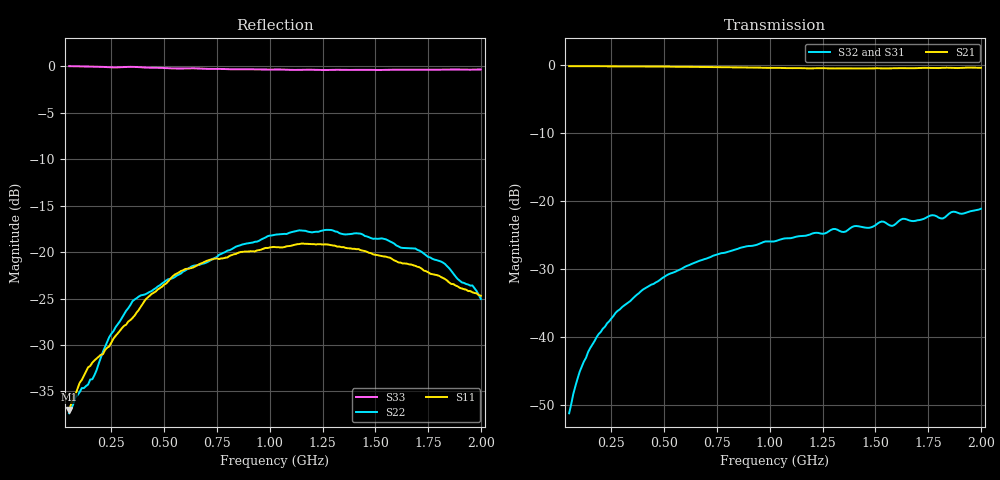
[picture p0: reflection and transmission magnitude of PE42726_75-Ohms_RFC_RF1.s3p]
! Created Wed Feb  7 16:17:06 2024
# hz S db R 75
! 3 Port Network Data from Sweep2.SP1.SP block
! freq  dbS11  angS11  dbS12  angS12  dbS13  angS13
!  dbS21  angS21
!  dbS22  angS22  dbS23  angS23
!  dbS31  angS31  dbS32  angS32
!  dbS33  angS33
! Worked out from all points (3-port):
!   196 points, 50 MHz to 2 GHz, reference 75 ohm
!   strongest paths, dB at 50 MHz, 540 MHz, 1.03 GHz, 1.52 GHz, 2 GHz:
!     S21: -0.1, -0.2, -0.4, -0.4, -0.4
!     S32: -51.2, -30.5, -25.8, -23.1, -21.1
!     S31: -50.9, -30.5, -25.9, -23.4, -21.2
!   lowest |S11| = -37.0 dB at 50 MHz (marker M1), VSWR 1.03, Z = 76.9 - j1.04 ohm
!   |S11| at or under -10 dB: start of sweep to end of sweep
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5e7  -36.97 -28.5  -0.11 -0.9  -51.13 85.0
     -0.11 -0.9  -37.35 -36.8  -50.62 85.8
     -50.91 87.5  -51.16 85.7  -0.00 -7.9
1.2e8  -33.31 -46.8  -0.12 -2.1  -43.20 85.2
       -0.12 -2.1  -34.64 -66.6  -43.46 82.2
       -43.34 86.1  -43.54 81.2  -0.03 -18.7
2.1e8  -30.99 -58.7  -0.13 -3.7  -38.48 83.8
       -0.13 -3.7  -30.74 -105.2  -38.75 76.8
       -38.46 83.1  -38.71 76.7  -0.08 -32.6
5.3e8  -22.88 -79.2  -0.19 -9.3  -30.67 74.0
       -0.19 -9.3  -22.86 -150.8  -30.69 56.3
       -30.59 73.6  -30.60 56.0  -0.24 -82.8
7.6e8  -20.76 -77.2  -0.26 -13.1  -27.80 67.3
       -0.25 -13.2  -20.29 174.2  -27.74 41.7
       -27.77 66.9  -27.69 41.1  -0.30 -119.0
1.03e9  -19.48 -81.8  -0.37 -17.2  -25.78 60.6
        -0.36 -17.3  -18.12 141.7  -25.69 24.9
        -25.94 60.5  -25.82 24.6  -0.37 -160.2
1.3e9  -19.30 -83.1  -0.43 -21.2  -24.45 55.5
       -0.45 -21.0  -17.68 112.8  -24.06 9.6
       -24.50 57.4  -24.06 11.2  -0.40 160.6
1.57e9  -20.61 -81.2  -0.42 -24.6  -23.40 53.2
        -0.44 -24.8  -18.87 82.3  -23.54 -2.9
        -23.38 54.3  -23.54 -1.4  -0.39 124.1
1.8e9  -22.54 -71.2  -0.37 -28.3  -22.51 52.4
       -0.39 -28.2  -20.94 52.8  -22.62 -10.5
       -22.24 52.4  -22.38 -10.5  -0.38 94.7
2e9  -24.71 -40.1  -0.32 -31.6  -21.59 52.5
     -0.35 -31.5  -25.06 28.2  -21.51 -17.5
     -21.17 51.3  -21.08 -18.8  -0.36 70.2
